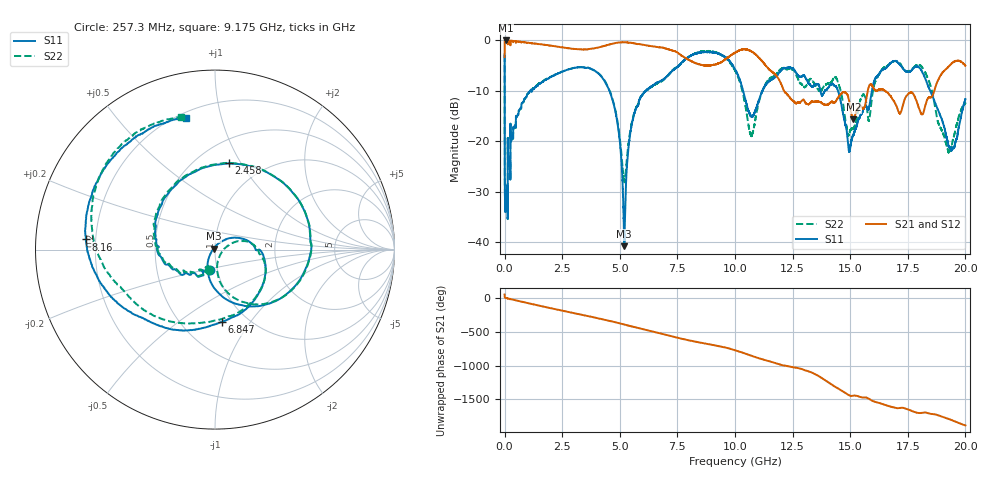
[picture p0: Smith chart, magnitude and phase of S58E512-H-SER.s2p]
!{S58E512}
!Johanson Technology Inc.
!www.johansontechnology.com
!Test Board Conditions:
!Substrate Type  RO4350B
!Substrate Thickness  60 mil
!Substrate Dk  3.66
!TL Type: GCPW
!TL Trace Width  115 mil
!TL Gap  52 mil
!Electrode orientation  Horizontal
!DUT TOPOLOGY	SERIES
!Mounting Pad LxW  55x428 mil
! Created Wed Apr 14 11:56:23 2021
# mhz S ma R 50
! 2 Port Network Data from SP1.SP block
! freq  magS11  angS11  magS21  angS21  magS12  angS12  magS22  angS22
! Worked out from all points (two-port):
!   20001 points, 300 kHz to 20 GHz, reference 50 ohm
!   highest |S21| = 0.00 dB at 43.3 MHz (marker M1); lowest = -15.6 dB at 15.14 GHz (marker M2)
!   |S21| within 3 dB of the highest: 398.1 kHz to 7.677 GHz (7.677 GHz wide, 200 % of centre); 9.809 GHz to 10.95 GHz (1.142 GHz wide, 11 % of centre)
!   lowest |S11| = -40.8 dB at 5.193 GHz (marker M3), VSWR 1.02, Z = 49.2 + j0.431 ohm
!   |S11| at or under -10 dB: 4.551 GHz to 6.131 GHz (1.581 GHz wide, 29.6 % of centre); 14.48 GHz to 15.94 GHz (1.466 GHz wide, 9.64 % of centre); 18.48 GHz to end of sweep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
!   |S22| runs from -35.5 to -2.1 dB; largest |S21 - S12| = 0.012
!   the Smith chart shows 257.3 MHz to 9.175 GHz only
!   S11 on the Smith chart (normalised r, x): 257.3 MHz: 0.92, -0.21; 2.458 GHz: 0.70, +0.89; 6.847 GHz: 0.77, -0.74; 8.16 GHz: 0.16, +0.04; 9.175 GHz: 0.23, +0.78
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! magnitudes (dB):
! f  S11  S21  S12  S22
! 300 kHz  -2.8  -3.3  -3.3  -2.9
! 43.3 MHz  -33.7  0.0  0.0  -33.7
! 105.3 MHz  -29.3  0.0  0.0  -29.2
! 257.3 MHz  -18.6  -0.2  -0.1  -18.6
! 2.458 GHz  -6.3  -1.3  -1.3  -6.3
! 3.334 GHz  -5.3  -1.8  -1.8  -5.3
! 4.645 GHz  -11.2  -0.7  -0.7  -11.1
! 5.193 GHz  -40.8  -0.4  -0.4  -28.0
! 5.627 GHz  -14.5  -0.6  -0.6  -14.4
! 6.667 GHz  -8.3  -1.3  -1.3  -8.4
! 6.847 GHz  -7.9  -1.4  -1.4  -8.0
! 8.16 GHz  -2.8  -4.2  -4.2  -2.8
! 9.175 GHz  -2.5  -4.7  -4.8  -2.4
! 10 GHz  -5.7  -2.5  -2.5  -6.0
! 10.71 GHz  -15.1  -2.2  -2.2  -19.0
! 11.52 GHz  -8.0  -5.9  -6.0  -7.6
! 13.33 GHz  -9.1  -12.1  -12.0  -7.9
! 15.14 GHz  -18.8  -15.6  -15.5  -17.6
! 16.67 GHz  -4.9  -10.6  -10.6  -4.9
! 18.14 GHz  -6.4  -14.7  -14.6  -5.5
! 19.28 GHz  -21.0  -5.1  -5.1  -22.3
! 20 GHz  -11.7  -5.0  -4.9  -12.4
